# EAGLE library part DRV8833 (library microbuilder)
DRV8833 Dual H-Bridge Motor Driver -- HTSSOP Package
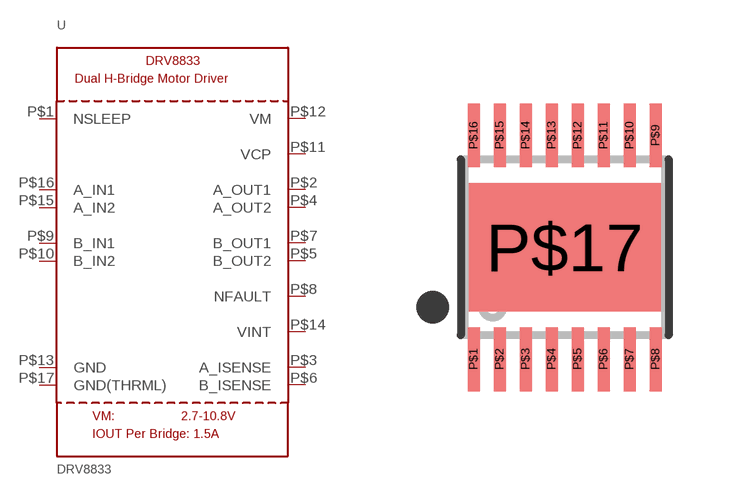
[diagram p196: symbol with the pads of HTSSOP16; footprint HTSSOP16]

Designator prefix U

## DRV8833  [HTSSOP16]
P$1  NSLEEP  in
P$2  A_OUT1  out
P$3  A_ISENSE
P$4  A_OUT2  out
P$5  B_OUT2  out
P$6  B_ISENSE
P$7  B_OUT1  out
P$8  NFAULT
P$9  B_IN1  in
P$10  B_IN2  in
P$11  VCP
P$12  VM  pwr
P$13  GND  pwr
P$14  VINT  pwr
P$15  A_IN2  in
P$16  A_IN1  in
P$17  GND(THRML)  pwr

## Footprint HTSSOP16 (pad centres in mm)
HTSSOP 16 (5x4.4mm 0.65mm Pitch) Source: http://www.ti.com/lit/ds/slvsar1b/slvsar1b.pdf
smd 0.3 x 1.6: P$1 -2.275,-2.8; P$2 -1.625,-2.8; P$3 -0.975,-2.8; P$4 -0.325,-2.8; P$5 0.325,-2.8; P$6 0.975,-2.8; P$7 1.625,-2.8; P$8 2.275,-2.8; P$9 2.275,2.8; P$10 1.625,2.8; P$11 0.975,2.8; P$12 0.325,2.8; P$13 -0.325,2.8; P$14 -0.975,2.8; P$15 -1.625,2.8; P$16 -2.275,2.8
smd 4.8 x 3.2: P$17 0,0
